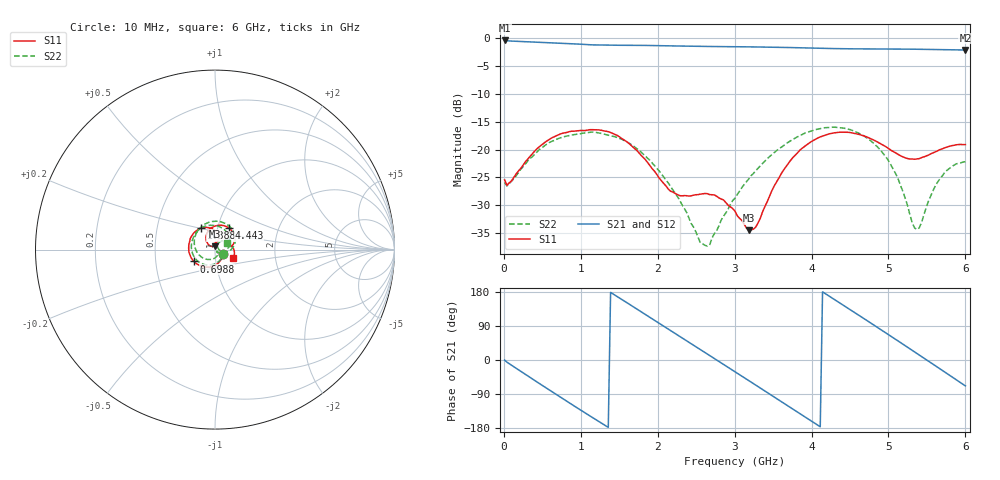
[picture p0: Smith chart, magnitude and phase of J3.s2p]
!Agilent Technologies,E8364B,MY43040528,A.07.50.67
!Agilent E8364B: A.07.50.67
!Date: Sunday, September 28, 2025 22:29:56
!Correction: S11(Full 2 Port(1,2))
!S21(Full 2 Port(1,2))
!S12(Full 2 Port(1,2))
!S22(Full 2 Port(1,2))
!S2P File: Measurements: S11, S21, S12, S22:
# Hz S  dB  R 50
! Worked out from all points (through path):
!   201 points, 10 MHz to 6 GHz, reference 50 ohm
!   highest |S21| = -0.44 dB at 10 MHz (marker M1); lowest = -2.2 dB at 6 GHz (marker M2)
!   group delay of S21, straight-line fit = 363 ps
!   lowest |S11| = -34.4 dB at 3.185 GHz (marker M3), VSWR 1.04, Z = 49.7 + j1.87 ohm
!   |S11| at or under -10 dB: start of sweep to end of sweep
!   |S22| runs from -37.3 to -16.0 dB; largest |S21 - S12| = 0.0076
!   S11 on the Smith chart (normalised r, x): 10 MHz: 1.10, -0.06; 698.9 MHz: 0.78, -0.10; 1.388 GHz: 0.83, +0.20; 4.443 GHz: 1.13, +0.28; 6 GHz: 1.21, -0.12
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1e7  -25.43 -29.9  -0.44 -0.2  -0.48 0.1  -25.89 -31.4
3.694e8  -20.78 -95.7  -0.70 -49.8  -0.70 -49.8  -21.28 -102.7
6.9885e8  -17.43 -150.7  -0.91 -93.2  -0.91 -93.1  -18.07 -165.1
1.0283e9  -16.58 166.2  -1.14 -136.1  -1.14 -136.0  -17.06 142.8
1.3877e9  -16.94 122.8  -1.31 178.4  -1.30 178.5  -17.52 88.2
1.65725e9  -19.28 92.4  -1.31 143.8  -1.31 143.9  -19.11 47.8
2.01665e9  -25.06 70.3  -1.37 97.1  -1.37 97.2  -23.78 -2.9
2.31615e9  -28.29 82.8  -1.45 58.4  -1.45 58.5  -29.88 -41.8
2.6456e9  -27.90 85.4  -1.51 15.7  -1.51 15.8  -37.31 -39.5
3.005e9  -31.03 77.9  -1.57 -30.9  -1.56 -30.8  -28.71 -71.5
3.1847e9  -34.43 98.4  -1.59 -54.4  -1.59 -54.3  -25.24 -104.3
3.27455e9  -33.89 123.8  -1.61 -66.2  -1.61 -66.1  -23.79 -120.9
3.57405e9  -25.13 139.0  -1.67 -105.5  -1.67 -105.4  -19.89 -171.2
3.81365e9  -20.65 121.5  -1.75 -137.0  -1.75 -136.9  -17.74 151.0
4.0233e9  -18.36 100.9  -1.82 -164.5  -1.82 -164.3  -16.55 120.0
4.23295e9  -17.17 79.2  -1.88 168.1  -1.89 168.2  -16.04 90.4
4.4426e9  -16.89 57.8  -1.93 140.7  -1.93 140.8  -16.23 62.2
4.7421e9  -17.87 30.7  -1.96 101.3  -1.96 101.4  -18.11 23.9
5.01165e9  -19.92 14.5  -1.97 65.4  -1.97 65.6  -22.25 -6.1
5.37105e9  -21.68 14.2  -2.02 17.1  -2.02 17.3  -34.31 25.6
5.67055e9  -20.00 6.1  -2.08 -23.4  -2.08 -23.3  -25.22 55.9
6e9  -19.11 -25.9  -2.15 -68.3  -2.15 -68.2  -22.17 28.0
